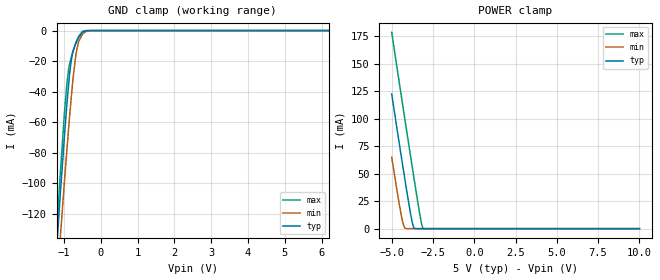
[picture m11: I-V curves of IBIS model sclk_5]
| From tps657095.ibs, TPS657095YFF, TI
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|   sclk_5 Model
[Model]   sclk_5
Model_type   Input
Vinl = 0.4
Vinh = 1.2
|   typ   min   max
|   (nom PVT)   (fast PVT)   (slow PVT)
C_comp   3.257e-12   3.234e-12   3.453e-12
| Where nom  PVT is Nominal Process, 5V, 27C
|   Fast PVT is Strong Process,  5.5V, -40C
|   Slow PVT is Weak Process,   4.5V, 125C
[Voltage Range]   5   4.5   5.5
|Junction Temperature
[Temperature Range]   27   125   -40
[Power Clamp Reference]   5   4.5   5.5
[GND Clamp Reference]   0   0   0
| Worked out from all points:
|   GND clamp passes 1 mA (typ) near -0.48 V on its own axis
|   POWER clamp passes 1 mA (typ) near -3.66 V on its own axis
[GND Clamp]
|   Voltage   I(typ)   I(min)   I(max)
-5V       -1.755A    -1.651A    -1.867A
-1.4V     -219.3mA   -239.9mA   -214.4mA
-1.184V   -138.6mA   -164.9mA   -127.2mA
-1.089V   -104.8mA   -133.1mA   -91.03mA
-990.5mV  -71.04mA   -100.8mA   -55.9mA
-919mV    -48.52mA   -78.4mA    -34.93mA
-869.5mV  -34.62mA   -63.49mA   -25.27mA
-805mV    -20.5mA    -45.19mA   -18.03mA
-670mV    -7.891mA   -15.08mA   -7.724mA
-599mV    -4.474mA   -7.097mA   -3.773mA
-473mV    -820.2uA   -1.871mA   -366.5uA
10V       0A         0A         0A
[POWER Clamp]
|   Voltage   I(typ)   I(min)   I(max)
-5V       122.6mA    64.98mA    178.6mA
-4.537V   77.05mA    21.91mA    132.4mA
-4.361V   60.14mA    7.872mA    115.1mA
-4.248V   49.4mA     1.76mA     104.1mA
-4.15V    40.09mA    159.3uA    94.43mA
-3.865V   14.26mA    150.8nA    66.64mA
-3.71V    2.889mA    0A         51.65mA
-3.61V    172.9uA    0A         42.06mA
-3.272V   0A         0A         10.96mA
-3.163V   0A         0A         2.802mA
-3.091V   0A         0A         279.9uA
10V       0A         0A         0A
